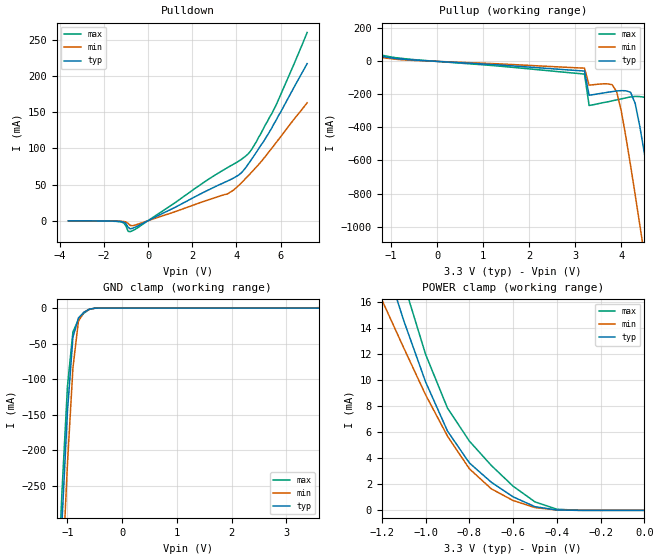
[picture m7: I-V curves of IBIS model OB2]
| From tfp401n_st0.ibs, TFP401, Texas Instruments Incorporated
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|   OUTPUT  MODEL
[Model]   OB2
Model_type   3-state
| variable   typ   min   max
C_comp   2pF   NA   NA
|   typ   min   max
[Temperature Range]   25.0   70   0
[Voltage range]   3.3V   3.0V   3.6V
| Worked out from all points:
|   slope of the pulldown table from 0 to 0.495 V, typ, clamps not added: 65.1 ohm
|   slope of the pullup table from 0 to 0.495 V, typ, clamps not added: 62.5 ohm
|   GND clamp passes 1 mA (typ) near -0.56 V on its own axis
|   POWER clamp passes 1 mA (typ) near -0.59 V on its own axis
[GND_clamp]
|Voltage   I(typ)   I(min)   I(max)
-3.6V     -5.15A     -5.23A     -5.11A
-1.2V     -475mA     -560mA     -431mA
-1.1V     -301mA     -384mA     -258mA
-1V       -145mA     -219mA     -110mA
-900mV    -40.7mA    -84.1mA    -33.4mA
-800mV    -14mA      -18.7mA    -16.4mA
-700mV    -5.9mA     -5.85mA    -7.15mA
-600mV    -1.53mA    -1.72mA    -1.77mA
-400mV    -10.7uA    -23.8uA    -8.94uA
3.6V      1.46uA     756uA      252pA
[Power_clamp]
|Note that the [Power_clamp] voltage table is referenced to Vcc
|and is calculated using Vtable=Vcc-Vmeasured.
|Voltage   I(typ)   I(min)   I(max)
-3.3V     145mA      102mA      188mA
-1.2V     19.9mA     16.2mA     23.9mA
-1.1V     14.6mA     12.5mA     17.5mA
-1V       9.88mA     8.89mA     12mA
-900mV    6.1mA      5.71mA     7.87mA
-800mV    3.65mA     3.2mA      5.33mA
-700mV    2.17mA     1.66mA     3.46mA
-600mV    1.04mA     756uA      1.86mA
-500mV    283uA      214uA      651uA
-400mV    28.7uA     27.2uA     87.1uA
-300mV    1.46uA     2.03uA     4.17uA
0V        235pA      318pA      252pA
[Pulldown]
|Voltage   I(typ)   I(min)   I(max)
-3.6V     -123uA     -85.6uA    -159uA
-1.3V     -955uA     -585uA     -1.34mA
-1.1V     -2.02mA    -1.09mA    -3.15mA
-900mV    -9.04mA    -3.61mA    -14.7mA
-800mV    -11.3mA    -6.62mA    -15.1mA
3.6V      54.9mA     37mA       73.4mA
4.1V      63.1mA     48.6mA     82.2mA
4.4V      72.5mA     57.8mA     88.8mA
4.6V      81.1mA     64.2mA     94.7mA
4.9V      94.5mA     74.1mA     109mA
5.8V      139mA      108mA      160mA
7.2V      217mA      163mA      260mA
[Pullup]
|Note that the [Pullup] voltage table is referenced to Vcc
|and is calculated using Vtable=Vcc-Vmeasured.
|Voltage   I(typ)   I(min)   I(max)
-3.3V     149mA      105mA      193mA
-1V       21.1mA     16.3mA     26.7mA
3.2V      -58.3mA    -41mA      -76.7mA
3.3V      -205mA     -144mA     -267mA
3.9V      -179mA     -185mA     -233mA
4.2V      -187mA     -630mA     -215mA
4.4V      -392mA     -989mA     -213mA
4.5V      -556mA     -1.17A     -217mA
4.6V      -730mA     -1.36A     -245mA
4.8V      -1.09A     -1.73A     -512mA
5.1V      -1.65A     -2.3A      -1.04A
6.6V      -4.56A     -5.23A     -3.92A
[Ramp]
|   typ   min   max
dV/dt_r   2.05v/900ps   1.87v/1.4ns   2.20v/600ps
dV/dt_f   1.95v/600ps   1.96v/1.1ns   2.08v/400ps
R_load = 5K
